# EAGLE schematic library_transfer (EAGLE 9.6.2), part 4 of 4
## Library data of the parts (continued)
U84 = ruark2:NCP781BMNADJTAGOSCT-ND: 150V 100mA Linear Voltage Regulator IC Positive Adjustable 1 Output 100mA 6-DFN (3.3x3.3); PARTNO: NCP781BMNADJTAGOSCT-ND
U85 = ruark2:NCP508SQ28T1G: Linear Voltage Regulator IC 1 Output 50mA SC-88A (SC-70-5/SOT-353); PARTNO: NCP508SQ28T1GOSCT-ND
U86 = ruark2:MTI-7-T: Accelerometer, Gyroscope, Magnetometer, 9 Axis Sensor I²C, SPI, UART Output; PARTNO: MTI-7-T-ND
U87 = ruark2:MPQ4436GRE-AEC1-Z: 45V 6A Buck Switching Regulator IC Positive Adjustable 0.815V 1 Output 20-PowerVFQFN; PARTNO: 1589-MPQ4436GRE-AEC1-ZCT-ND
U88 = ruark2:MP86952
U89 = ruark2:MP5515: Wide Input 2.7 - 18V, 5A, High-Efficiency Bidirectional, Power Back-Up Manager with Integrated Hot-Swap, I2C, ADC, and Cap Health Test
U90 = ruark2:MP3423: Boost Switching Regulator IC Positive Adjustable 2.5V 1 Output 9A (Switch) 14-PowerVFQFN; PARTNO: 1589-1171-1-ND
U91 = ruark2:MIC28516T-E/PHA: Switching Voltage Regulators 70V/8A Hyper Speed Control Synchronous DC/DC Buck Regulator with External Soft Start; PARTNO: 150-MIC28516T-E/PHACT-ND
U92 = ruark2:MIC7221YM5-TR: Comparator General Purpose Open Drain SOT-23-5; PARTNO: 576-2901-1-ND
U93 = ruark2:MIC4604YM-TR: Half-Bridge Gate Driver IC Non-Inverting 8-SOIC, 85V, 1A; PARTNO: 576-4396-1-ND
U94 = ruark2:MIC2920A-12WS: Linear Voltage Regulator IC Positive Fixed 1 Output 12V 400mA SOT-223; PARTNO: 576-1750-5-ND
U95 = ruark2:MIC2288: Boost Switching Regulator IC Positive Adjustable 2.5V 1 Output 1.2A (Switch) SOT-23-5 Thin, TSOT-23-5, IN 2.5-10, OUT 2.5-34; PARTNO: 576-1729-1-ND
U96 = ruark2:MIC2176-1YMM: Buck Regulator Positive Output Step-Down DC-DC Controller IC 10-MSOP 4.5-65V Synchronous; PARTNO: 576-3756-5-ND
U97 = ruark2:MIC842LYC5-TR: Comparator with Voltage Reference Push-Pull SC-70-5 Active High
U98 = ruark2:ME6211C12M5G-N: 300mA 70dB@(1kHz) Fixed 1.2V Positive electrode 6.5V SOT-23-5 Linear Voltage Regulators (LDO) ROHS; JLCPCB: C236672
U99 = ruark2:MCP73832T-5ACI/OT: Charger IC Lithium Ion/Polymer SOT-23-5 450mA; PARTNO: MCP73832T-5ACI/OTCT-ND
U100 = ruark2:MCP73811T-420I/OT: Charger IC Lithium Ion/Polymer SOT-23-5 450mA; PARTNO: MCP73811T-420I/OTCT-ND
U101 = ruark2:MCP73114-0NSI/MF: Charger IC Lithium Ion/Polymer 10-DFN (3x3); PARTNO: MCP73114-0NSI/MF-ND
U102 = ruark2:MCP23017: I/O Expander 16 CH, I²C 1.7MHz 28-SSOP; PARTNO: MCP23017T-E/SSCT-ND
U103 = ruark2:MCP9700: Temperature Sensor Analog, Local -40°C ~ 125°C 10mV/°C SOT-23-3; PARTNO: MCP9700T-E/TTCT-ND
U104 = ruark2:MCP6561T-E/OTVAO: Comparator General Purpose CMOS, Push-Pull, Rail-to-Rail, TTL SOT-23-5, 800ns, 5mVh; PARTNO: 150-MCP6561T-E/OTVAOCT-ND
U105 = ruark2:MCP6549-I/ST: Comparator General Purpose CMOS, 1uA power, 10pA bias, 7mV offset, Open-Drain, Rail-to-Rail, TTL 14-TSSOP; PARTNO: MCP6549-I/ST-ND
U106 = ruark2:MCP6542T-I/SN: Comparator General Purpose CMOS, Push-Pull, Rail-to-Rail, TTL 8-SOIC; PARTNO: MCP6542T-I/SNCT-ND
U107 = ruark2:MCP4725A1T-E/CH: 12 Bit Digital to Analog Converter 1 SOT-23-6 DAC I2C; PARTNO: MCP4725A1T-E/CHCT-ND
U108 = ruark2:MCP1702T-5002E/CB: Linear Voltage Regulator IC Positive Fixed 1 Output 250mA SOT-23A-3; PARTNO: MCP1702T-5002E/CBCT-ND
U109 = ruark2:MCP1665T-E/MRA: Boost Switching Regulator IC Positive Adjustable 2.8V 1 Output 1A 10-VFQFN Exposed Pad; PARTNO: MCP1665T-E/MRACT-ND
U110 = ruark2:MCP1632-BAE/MS: Boost, Cuk, Flyback, SEPIC Regulator Positive Output Step-Up, Step-Up/Step-Down DC-DC Controller IC 8-MSOP; PARTNO: MCP1632-BAE/MS-ND
U111 = ruark2:MCP1407-E/SN: Low-Side Gate Driver IC Non-Inverting 8-SOIC, 6A; PARTNO: MCP1407-E/SN-ND
U112 = ruark2:MCP6L01T-E/OT: General Purpose Amplifier 1 Circuit Rail-to-Rail SOT-23-5; PARTNO: MCP6L01T-E/OTCT-ND
U113 = ruark2:MC14044BDR2G: THIS PN HAS INVERED INPUTS S-R Latch 4 Channel 1:1 IC Tri-State 16-SOIC; PARTNO: MC14044BDR2GOSCT-ND
U114 = ruark2:MC14043BDR2G: IC LATCH R-S QUAD P/N 16-SOIC; PARTNO: MC14043BDR2GOSCT-ND
U115 = ruark2:MC74LVX08DTR2G: Quad 2-Input AND Gate AND Gate IC 4 Channel 14-TSSOP; MPN: MC74LVX08DTR2G; OC_FARNELL: 1353762; OC_NEWARK: 26K4279; PACKAGE: TSSOP-14; PARTNO: MC74LVX08DTR2GOSCT-ND; SUPPLIER: On Semiconductor
U116 = ruark2:MAX9107: Comparator General Purpose TTL 8-SOIC; PARTNO: MAX9107ESA+-ND
U117 = ruark2:MAX9095ASD+: Comparator General Purpose Open Drain 14-SOIC; PARTNO: MAX9095ASD+-ND
U118 = ruark2:MAX5084ATT+T: 65V Linear Voltage Regulator IC Positive Adjustable (Fixed) 1 Output 200mA 6-TDFN-EP (3x3); PARTNO: MAX5084ATT+CT-ND
U119 = ruark2:MAX3232ECDR: 3.3V 2/2 Transceiver Full RS232 16-SOIC; PARTNO: 296-19851-1-ND
U120 = ruark2:MAX2680AUT+T: RF Mixer IC Cellular, ISM, PCS, WLL Down Converter 400MHz ~ 2.5GHz SOT-23-6; PARTNO: MAX2680AUT+T-ND
U121 = ruark2:MAX2671EUT+T: RF Mixer IC Cellular, ISM, PCS, WLAN Up Converter 400MHz ~ 2.5GHz SOT-6; PARTNO: MAX2671EUT+TCT-ND
U122 = ruark2:MAX2663EUT+T: RF Mixer IC Cellular, ISM, PCS, WLAN Up Converter 400MHz ~ 2.5GHz SOT-23-6; PARTNO: MAX2663EUT+T-ND
U123 = ruark2:MAX232: 2/2 Transceiver Full RS232 16-SOIC; PARTNO: 296-26141-1-ND
U124 = ruark2:MAX-M8Q-0: MAX-M8 RF Receiver BeiDou, Galileo, GLONASS, GNSS, GPS 1.575GHz -167dBm; PARTNO: 672-MAX-M8Q-0CT-ND
U125 = ruark2:LTV827S-TA1: Optoisolator Transistor Output 5000Vrms 2 Channel 8-SMD; PARTNO: 160-2040-1-ND
U126 = ruark2:LTV-816S: Optoisolator Transistor Output 5000Vrms 1 Channel 4-SMD; PARTNO: 160-1892-1-ND
U127 = ruark2:LTC6993CS6-1#TRMPBF: Fixed Pulse Generator Monostable Multivibrator 11ns TSOT-23-6; PARTNO: LTC6993CS6-1#TRMPBFCT-ND
U128 = ruark2:LTC6992CS6-1#TRMPBF: Oscillator, Silicon IC 3.81Hz ~ 1MHz TSOT-23-6; PARTNO: LTC6992CS6-1#TRMPBFCT-ND
U129 = ruark2:LTC6990CS6#TRMPBF: VCO Oscillator, Silicon IC 488Hz ~ 1MHz TSOT-23-6; PARTNO: LTC6990CS6#TRMPBFCT-ND
U130 = ruark2:LTC4365: Overvoltage, Undervoltage and Reverse Supply Protection Controller Charge Pump, -40 to +60V
U131 = ruark2:LT8410IDC#TRMPBF: Boost Switching Regulator IC Positive Adjustable 1.235V 1 Output 20mA (Switch) 8-WFDFN Exposed Pad; PARTNO: LT8410IDC#TRMPBFCT-ND
U132 = ruark2:LT6654BHS6-2.5#TRMPBF: 2.5V Series Voltage Reference IC ±0.1% TSOT-23-6; PARTNO: LT6654BHS6-2.5#TRMPBFCT-ND
U133 = ruark2:LT3088EDD#PBF: Linear Voltage Regulator IC Positive Adjustable 36V 1 Output 800mA 8-DFN (3x3); PARTNO: LT3088EDD#PBF-ND
U134 = ruark2:LT3080: Linear Voltage Regulator IC Positive Adjustable 1 Output 0 V ~ 36 V 1.1A SOT-223-3; PARTNO: LT3080EST#TRPBFCT-ND
U135 = ruark2:LT3012EFETRPBF: 60V 250mA LDO Linear Voltage Regulator IC Positive Adjustable 1 Output 16-TSSOP-EP; PARTNO: LT3012EFE#TRPBFCT-ND
U136 = ruark2:LT1678: General Purpose Amplifier 2 Circuit Rail-to-Rail 8-SO 20MHz Rail to Rail; PARTNO: LT1678CS8#TRPBFCT-ND
U137 = ruark2:LT1054: Charge Pump Switching Regulator IC Positive or Negative Adjustable (Fixed) 3.5V (-Vin, 2Vin) 1 Output 100mA 16-SOIC (0.295", 7.50mm Width); PARTNO: 296-17595-1-ND
U138 = ruark2:LP28013A: TDFN-10 Battery Management ICs ROHS JLCPCB: C517139
U139 = ruark2:LMV7219M5X: Comparator General Purpose Push-Pull, Rail-to-Rail SOT-23-5 (OPA320 pinout compatible); PARTNO: LMV7219M5X-ND
U140 = ruark2:LMV321IDBVR: General Purpose Amplifier 1 Circuit Rail-to-Rail SOT-23-5; PARTNO: 296-9567-1-ND
U141 = ruark2:LMT87LPG: Temperature Sensor Analog, Local -50°C ~ 150°C 13.6mV/°C TO-92S; PARTNO: 296-47011-ND
U142 = ruark2:LMR38020SDDAR: Buck Switching Regulator IC Positive Adjustable 1V 1 Output 2A 8-PowerSOIC (0.154", 3.90mm Width); PARTNO: 296-LMR38020SDDARCT-ND
U143 = ruark2:LMP2231: General Purpose Amplifier 1 Circuit Rail-to-Rail SOT-23-5, 0.02pA, 10uV
U144 = ruark2:LMC7660: Charge Pump Switching Regulator IC Negative Fixed -Vin 1 Output 8-SOIC (0.154", 3.90mm Width); PARTNO: LMC7660IMX/NOPBCT-ND
U145 = ruark2:LMC662CN/NOPB: SURFACE MOUNT DIP SOCKET FOR: LMC662CN/NOPB CMOS Amplifier 2 Circuit Push-Pull, Rail-to-Rail 8-PDIP | PURCHASE 110-87-308-41-105191; PARTNO: LMC662CN/NOPB-ND
U146 = ruark2:LMC662CMX/NOPB: CMOS Amplifier 2 Circuit Push-Pull, Rail-to-Rail 8-SOIC; PARTNO: 296-36891-1-ND
U147 = ruark2:LMC555CMM/NOPB: 555 Type, Timer/Oscillator (Single) IC 2.1MHz 8-SOIC; PARTNO: LMC555CMM/NOPBCT-ND
U148 = ruark2:LM46002AQPWPRQ1: Buck Switching Regulator IC Positive Adjustable 1V 1 Output 2A 16-TSSOP (0.173", 4.40mm Width) Exposed Pad 60V; PARTNO: 296-48923-1-ND
U149 = ruark2:LM25116MHX/NOPB: Buck Regulator Positive Output Step-Down DC-DC Controller IC 20-HTSSOP; PARTNO: 296-35258-1-ND
U150 = ruark2:LM7301: General Purpose Amplifier 1 Circuit Rail-to-Rail SOT-23-5; PARTNO: LM7301IM5X/NOPBCT-ND
U151 = ruark2:LM5155: Boost, Flyback, SEPIC Regulator Positive Output Step-Up, Step-Up/Step-Down DC-DC Controller IC 12-WSON (3x2); PARTNO: 296-LM5155DSSRCT-ND
U152 = ruark2:LM5134-SOT: Low-Side Gate Driver IC Inverting, Non-Inverting SOT-23-6 7.6A; PARTNO: 296-40244-1-ND
U153 = ruark2:LM5102MM/NOPB: IC GATE DRVR HALF-BRIDGE 10VSSOP; PARTNO: LM5102MM/NOPBCT-ND
U154 = ruark2:LM4040DYM3-2.5-TR: Shunt Voltage Reference IC ±1% 15mA SOT-23-3; PARTNO: 576-1047-1-ND
U155 = ruark2:LAN9512: Ethernet Bridge, USB to Ethernet USB 2.0, 10/100 Base-T/TX PHY USB Interface 64-QFN (9x9); PARTNO: 638-1086-ND
U156 = ruark2:LAN8742A-CZ-TR: 1/1 Transceiver Ethernet 24-SQFN (4x4); PARTNO: LAN8742A-CZ-CT-ND
U157 = ruark2:L6491: Half-Bridge Gate Driver IC Non-Inverting 14-SO 4A; PARTNO: 497-15443-5-ND
U158 = ruark2:L5150BNTR: Linear Voltage Regulator IC 40 Vin Positive Output 5V 150mA SOT-223; PARTNO: 497-11659-1-ND
U159 = ruark2:L4931: Linear Voltage Regulator IC Positive Fixed 1 Output 5V 250mA 8-SO; PARTNO: 497-1156-1-ND
U160 = ruark2:L78M05ABDT-TR: 62dB@(120Hz) 500mA Fixed 5V Positive 35V TO-252 Linear Voltage Regulators (LDO) ROHS; PARTNO: C58069
U161 = ruark2:K78U05-500R3: Non-Isolated PoL Module DC DC Converter 1 Output 5V 500mA 9V - 90V Input; PARTNO: 2725-K78U05-500R3-ND
U162 = ruark2:ISO1640BDR: I²C Digital Isolator 3000Vrms 2 Channel 50kV/µs CMTI 8-SOIC (0.154", 3.90mm Width); PARTNO: 296-ISO1640BDRCT-ND
U163 = ruark2:ISL83490IBZ-T: 1/1 Transceiver Full RS422, RS485 8-SOIC 3.3V; PARTNO: ISL83490IBZ-TCT-ND
U164 = ruark2:ISL21080DIH312Z-TK: Series Voltage Reference IC 1.25V ±0.6% 7mA SOT-23-3; PARTNO: ISL21080DIH312Z-TKCT-ND
U165 = ruark2:IRS2304SPBF: Half-Bridge Gate Driver IC Non-Inverting 8-SOIC 600V 290mA; PARTNO: IRS2304SPBF-ND
U166 = ruark2:IRS2186: Half-Bridge Gate Driver IC Non-Inverting 8-SOIC; PARTNO: IRS2186SPBF-ND
U167 = ruark2:IRM-05-5: Enclosed AC DC Converters 1 Uitgang 5V 1A 85 ~ 305 VAC, 120 ~ 430 VDC Input; PARTNO: 1866-3027-ND
U168 = ruark2:INA240A3PW: –4-V to 80-V, Bidirectional, Ultra-Precise Current Sense Amplifier With Enhanced PWM Rejection
U169 = ruark2:INA210CIDCKR: Current Sense Amplifier 1 Circuit SC-70-6 200V/V; PARTNO: 296-48548-1-ND
U170 = ruark2:INA195AIDBVR: 100 V/V, 3%, 80V, Current Monitor Regulator High-Side SOT-23-5; PARTNO: 296-26067-1-ND
U171 = ruark2:INA181A3IDBVR: Current Sense Amplifier 1 Circuit Rail-to-Rail SOT-23-6; PARTNO: 296-47658-1-ND
U172 = ruark2:INA180A3IDBVR: Current Sense Amplifier 1 Circuit Rail-to-Rail SOT-23-5 High/Low side 100V/V; PARTNO: 296-47654-1-ND
U173 = ruark2:HTCC-AB01: HTCC-AB01
U174 = ruark2:HMC544A: RF Switch IC WiMax, WLAN SPDT 4GHz 50 Ohm SOT-26; PARTNO: 1127-3066-ND
U175 = ruark2:HMC385LP4E: VCO 2.25GHz ~ 2.5GHz 24-QFN (4x4); PARTNO: 1127-1357-ND
U176 = ruark2:HELTEC_WIFI_LORA_32_V3
U177 = ruark2:HEF4052B: Dual 4 Channel Analog Multiplexer; PARTNO: 1727-6411-1-ND
U178 = ruark2:HD3SS3412ARUAT: PCI Express® Switch IC 4 Channel 42-WQFN (3.5x9.0); PARTNO: 296-HD3SS3412ARUATCT-ND
U179 = ruark2:HCF4010YM013TR: Voltage Level Translator Unidirectional 6 Circuit 1 Channel 16-SO; PARTNO: 497-13665-1-ND
U180 = ruark2:GVA-84+: RF Amplifier IC CATV, DBS, LTE, MMDS, Wireless LAN 0Hz ~ 7GHz SOT-89; PARTNO: 3157-GVA-84+CT-ND
U181 = ruark2:FT232RL: USB Bridge, USB to UART USB 2.0 UART Interface 28-SSOP FTDI; PARTNO: 768-1007-1-ND
U182 = ruark2:FM2113: SOT-23-6 Battery Protection UVLO, OV, OC
U183 = ruark2:FAN3180: Low-Side Gate Driver IC Non-Inverting SOT-23-5 2A; PARTNO: FAN3180TSXCT-ND
U184 = ruark2:FAN3111ESX: 1.4A, Low-Side Gate Driver IC Non-Inverting SOT-23-5; PARTNO: FAN3111ESXCT-ND
U185 = ruark2:EL5171: Single Ended to Differential Amplifier 1 Circuit 8-SOIC; PARTNO: EL5171ISZ-ND
U186 = ruark2:DS1100Z-500: Delay Line IC Nonprogrammable 5 Tap 500ns 8-SOIC (0.154", 3.90mm Width); PARTNO: DS1100Z-500+-ND
U187 = ruark2:DS18S20: Temperature Sensor Digital, Local -55°C ~ 125°C 8 b TO-92-3; PARTNO: DS18S20+-ND
U188 = ruark2:DRV8231ADDAR: 33V, 3.7A, Bipolar Motor Driver NMOS PWM 8-SO PowerPad 2 H-BRIDGE; PARTNO: 296-DRV8231ADDARCT-ND
U189 = ruark2:DP83822IRHBR: 10/100 Ethernet PHY RGMII/RMII/MII; PARTNO: 296-44794-1-ND
U190 = ruark2:DP83TD510ERHBR: 1/1 Transceiver 10BASE-T1L IEEE 802.3 32-VQFN (5x5); PARTNO: 296-DP83TD510ERHBRCT-ND
U191 = ruark2:DAC5571IDBVR: 8 Bit Digital to Analog Converter 1 SOT-23-6; PARTNO: 296-38918-1-ND
U192 = ruark2:COM13025-48.000-T-TR: 48 MHz XO (Standard) HCMOS Oscillator 3.3V Enable/Disable 4-SMD, No Lead; PARTNO: 2151-COM13025-48.000-T-TRCT-ND
U193 = ruark2:CO32H4-25.000-33GDTST: 3.3V~3.3V ±50ppm 25MHz HCMOS SMD3225-4P Oscillators ROHS 4-SMD, No Lead
U194 = ruark2:CM108: CM108 USB Audio
U195 = ruark2:CD40257: Multiplexer 4 x 1:2 16-SOIC; PARTNO: 296-32875-5-ND
U196 = ruark2:CD74HC4017M96: Counter IC Counter, Decade 1 Element 10 Bit Positive Edge 16-SOIC 35MHz; PARTNO: 296-12808-1-ND
U197 = ruark2:CBTL02042ABQ,115: DisplayPort, PCIe, USB Switch IC 2 Channel 20-DHVQFN (4.5x2.5); PARTNO: 568-6676-1-ND
U198 = ruark2:BQ7790512PWR: 3-5S Stackable to 20S Battery protection IC. 2.8V to 4.175V; PARTNO: 296-50465-1-ND
U199 = ruark2:BQ24616
U200 = ruark2:BQ24171: Charger IC Lithium Ion/Polymer 24-VQFN (5.5x3.5); PARTNO: 296-41205-1-ND
U201 = ruark2:BNO080: Accelerometer, Gyroscope, Magnetometer, 9 Axis Sensor I²C, SPI, UART Output; PARTNO: 1888-1000-1-ND
U202 = ruark2:BMP280: Pressure Sensor 4.35PSI ~ 15.95PSI (30kPa ~ 110kPa) Absolute 16b 8-SMD; PARTNO: 828-1064-1-ND
U203 = ruark2:BGU8051: RF Amplifier IC GSM, LTE, W-CDMA 300MHz ~ 1.5GHz 8-HWSON (2x2); PARTNO: 568-BGU8051XCT-ND
U204 = ruark2:BGU6102,147: RF Amplifier 40MHz - 4GHz, P1dB =9.5dBm, G=19dB, NF=2.3dB, I=20mA, V=1.5-5V, 6-HXSON (1.3x2); PARTNO: 568-10150-1-ND
U205 = ruark2:BGB741L7ESDE6327XTSA1: RF Amplifier IC Cellular, RKE, WiFi 50MHz ~ 3.5GHz PG-TSLP-7-1, NF=1dB, P1dB= -6.6dBm; PARTNO: BGB741L7ESDE6327XTSA1CT-ND
U206 = ruark2:BGA2869,115: RF Amplifier IC General Purpose 0Hz ~ 2.2GHz 6-TSSOP; PARTNO: 568-8535-1-ND
U207 = ruark2:BGA2866,115: RF Amplifier 0Hz - 2.2GHz, P1dB=3dBm, G=24.3dB, NF=3.9, I=17.4mA, V=5V, 6-TSSOP; PARTNO: 568-6213-1-ND
U208 = ruark2:BGA427H6327XTSA1: RF Amplifier 0Hz - 3GHz, G=18.5 dB, NF= 2.2dB, I= 25mA, V=2-5V, PG-SOT343-4; PARTNO: BGA427H6327XTSA1CT-ND
U209 = ruark2:BD9C401EFJ-E2: Buck Switching Regulator IC Positive Adjustable 0.8V 1 Output 4A 8-SOIC (0.154", 3.90mm Width) Exposed Pad; PARTNO: 846-1116-1-ND
U210 = ruark2:B39921B2672P810: 915MHz Frequency General Purpose RF SAW Filter (Surface Acoustic Wave) 1.1dB 26MHz Bandwidth 5-SMD, No Lead; PARTNO: 1752-B39921B2672P810CT-ND
U211 = ruark2:B39431B3710U410: 433.92MHz Frequency Remote Control RF SAW Filter (Surface Acoustic Wave) 2dB 1.7MHz Bandwidth 6-SMD, No Lead
U212 = ruark2:AX5043: IC RF TxRx Only General ISM < 1GHz 27MHz ~ 1.05GHz 28-VFQFN Exposed Pad; PARTNO: AX5043-1-TA05OSCT-ND
U213 = ruark2:ATTINY85V-10SUR: AVR AVR® ATtiny, Functional Safety (FuSa) Microcontroller IC 8-Bit 10MHz 8KB (4K x 16) FLASH 8-SOIC; PARTNO: ATTINY85V-10SURCT-ND
U214 = ruark2:ATA6561-GAQW-N: 1/1 Transceiver CAN 8-SO; PARTNO: ATA6561-GAQW-NCT-ND
U215 = ruark2:AT2659: 1.4V~3.6V 4.3mA DFN-6(1x1.6) Low Noise Amplifiers (LNA) - RF ROHS; JLCPCB: C92450
U216 = ruark2:AP65550SP-13: Buck Switching Regulator IC Positive Adjustable 0.76V 1 Output 5A 8-SOIC (0.154", 3.90mm Width) Exposed Pad; PARTNO: AP65550SP-13DICT-ND
U217 = ruark2:AP9211SA: Battery Battery Protection IC Lithium-Ion U-DFN2030-6 (Type C); PARTNO: AP9211SA-AE-HAC-7DICT-ND
U218 = ruark2:AP2114H-3.3: Linear Voltage Regulator IC Positive Fixed 1 Output 3.3V 1A SOT-223; PARTNO: AP2114H-3.3TRG1DICT-ND
U219 = ruark2:AP2114H-2.5: Linear Voltage Regulator IC Positive Fixed 1 Output 2.5V 1A SOT-223; PARTNO: AP2114H-2.5TRG1DICT-ND
U220 = ruark2:AP2114H-1.8: Linear Voltage Regulator IC Positive Fixed 1 Output 1.8V 1A SOT-223; PARTNO: AP2114H-1.8TRG1DICT-ND
U221 = ruark2:AOZ128: Buck Switching Regulator IC Positive Adjustable 0.8V 1 Output 4A 8-SOIC (0.154", 3.90mm Width) Exposed Pad; PARTNO: 785-1689-1-ND
U222 = ruark2:AMS1117-3.3: 72dB@(120Hz) 1A Fixed 3.3V Positive electrode SOT-223-3 Linear Voltage Regulators (LDO) ROHS
U223 = ruark2:AG1170: Aliexpress SLIC
U224 = ruark2:ADS1115IDGSR: 16 Bit Analog to Digital Converter 2 Input 1 Sigma-Delta 10-VSSOP; PARTNO: 296-38849-1-ND
U225 = ruark2:ADP7142AUJZ-3.3-R7: 40V Linear Voltage Regulator IC Positive Fixed 3.3V 1 Output 200mA TSOT-23-5; PARTNO: ADP7142AUJZ-3.3-R7CT-ND
U226 = ruark2:ADG812YRUZ-REEL7: 4 Circuit IC Switch 1:1 650mOhm 16-TSSOP SPST; PARTNO: ADG812YRUZ-REEL7CT-ND
U227 = ruark2:ADF4351: IC SYNTH PLL VCO 32LFCSP; PARTNO: ADF4351BCPZ-RL7CT-ND
U228 = ruark2:ADF4118BRUZ: IC PLL FREQ SYNTHESIZER 16-TSSOP 3GHz; PARTNO: ADF4118BRUZ-ND
U229 = ruark2:AD8306: Limiting-Logarithmic Amplifier IC Receiver Signal Strength Indication (RSSI) 16-SO; PARTNO: AD8306ARZ-ND
U230 = ruark2:ACS781KLRTR-150B-T: Current Sensor 150A 1 Channel Hall Effect, Differential Bidirectional 7-PowerSMD Module. 3V3, 8.8mV/A; PARTNO: 620-1827-1-ND
U231 = ruark2:ACS711ELCTR-25AB-T: Current Sensor 25A 1 Channel Hall Effect, Open Loop Bidirectional 8-SOIC (0.154", 3.90mm Width); PARTNO: 620-1371-1-ND
U232 = ruark2:ACS711ELCTR-12AB-T: Current Sensor 12.5A 1 Channel Hall Effect, Open Loop Bidirectional 8-SOIC (0.154", 3.90mm Width), 5V; PARTNO: 620-1370-1-ND
U233 = ruark2:ACPL-782T-300E: Isolation Amplifier 1 Circuit Differential 8-DIP Gull Wing; PARTNO: 516-2337-5-ND
U234 = ruark2:0026605020: Connector Header Through Hole, Right Angle 2 position 0.156" (3.96mm); PARTNO: WM4640-ND
U235 = ruark2:74VHC4040FT: Counter IC Binary Counter 1 Element 12 Bit Negative Edge 16-TSSOP; PARTNO: 74VHC4040FTCT-ND
U236 = ruark2:74LVCH2T45DC,125: Voltage Level Translator Level Shifter Bidirectional 1 Circuit 2 Channel 420Mbps 8-VSSOP; PARTNO: 1727-4596-1-ND
U237 = ruark2:74LVC4245A: Voltage Level Translator Bidirectional 1 Circuit 8 Channel 24-TSSOP; PARTNO: 1727-4308-1-ND
U238 = ruark2:74HC4051D,653: 1 Circuit IC Switch 8:1 120Ohm 16-SO +/- 4V; PARTNO: 1727-2807-1-ND
U239 = ruark2:74AHC14PW,112: IC HEX SCHMITT-TRIG INV 14TSSOP; PARTNO: 296-1086-1-ND
U240 = ruark2:000: 1 Circuit IC Switch 8:1 75Ohm 16-SOIC; PARTNO: 296-3827-1-ND
U$1 = ruark2:ZF43610
U$2 = ruark2:XT30PW-F
U$3 = ruark2:WA-T247-101E: Heat Sink TO-247 Aluminum 1.0W @ 20°C Board Level, Vertical; PARTNO: WA-T247-101E-ND
U$4 = ruark2:VERT-55351
U$5 = ruark2:UA78M33CKVURG3: Linear Voltage Regulator IC 1 Output 500mA TO-252-3; PARTNO: 296-21208-1-ND
U$6 = ruark2:TRF37D73IDSGT: RF Amplifier IC 1MHz - 6GHz, P1dB=16.5dB, G=19.5dB, NF=3.2dB, 8-WSON (2x2); PARTNO: 296-38827-1-ND
U$7 = ruark2:TP65H035WS: N-Channel 650V 46.5A (Tc) 156W (Tc) Through Hole TO-247-3 WARNING: GATE-SOURCE-DRAIN!; PARTNO: TP65H035WS-ND
U$8 = ruark2:TOROID2
U$9 = ruark2:TOROID1
U$10 = ruark2:TDA21490
U$11 = ruark2:STW40N65M2: N-Channel 650V 32A (Tc) 250W (Tc) Through Hole TO-247; PARTNO: 497-15576-5-ND
U$12 = ruark2:SPU01M-05: Isolated Module DC DC Converter 1 Output 5V 200mA 10.8V - 13.2V Input; PARTNO: SPU01M-05
U$13 = ruark2:SP1312/S
U$14 = ruark2:SIP32408DNP-T1-GE4: Power Switch/Driver 1:1 N-Channel 3.5A 4-TDFN (1.2x1.6); PARTNO: SIP32408DNP-T1-GE4CT-ND
U$15 = ruark2:PLUG
U$16 = ruark2:PINHD20
U$17 = ruark2:PA1005.100NLT: 20A 1:100 Current Sense Transformer 50kHz ~ 1MHz 0.75 mOhm Primary, 5.5 Ohm Secondary 2mH Surface Mount; PARTNO: PA1005.100NLT
U$18 = ruark2:OLED
U$19 = ruark2:MC3417: Continuously Variable Slope Delta (CVSD) Modulator / Demodulator
U$20 = ruark2:LM25037: Full-Bridge, Half-Bridge, Push-Pull Regulator Positive, Isolation Capable Output Step-Up/Step-Down DC-DC Controller IC 16-TSSOP; PARTNO: 296-35257-1-ND
U$21 = ruark2:LM5134: Low-Side Gate Driver IC Inverting, Non-Inverting 6-WSON (3x3) 7.6A; PARTNO: 296-40245-1-ND
U$22 = ruark2:HMC313E: RF Amplifier IC HiperLAN, UNII, 0Hz - 6GHz, P1dB=14dBm, G=17dB, NF=6.5dB, I=50mA, V=5V, SOT-23-6; PARTNO: 1127-2932-ND
U$23 = ruark2:EPC2033: TRANS GAN 150V 7MOHM BUMPED DIE; PARTNO: 917-1131-1-ND
U$24 = ruark2:ECS-250-18-36B-CKY-TR: 25 MHz Crystal 10ppm; PARTNO: XC3051CT-ND
U$25 = ruark2:DS02C-254-1L-04BE: Dip Switch SPST 4 Position Through Hole, Right Angle Piano Actuator 25mA 24VDC; PARTNO: 2223-DS02C-254-1L-04BE-ND
U$26 = ruark2:CSAC
U$27 = ruark2:COUPLED_INDUCTOR2
U$28 = ruark2:COUPLED_INDUCTOR
U$29 = ruark2:CMZ5951CTR13: Zener Diode 120V 500mW ±5% Surface Mount SMA; PARTNO: CMZ5951BTR13CT-ND
U$30 = ruark2:BGA6589,135: RF Amplifier IC PCS, CDPD, Broadcast Television, 0Hz - 3GHz, P1dB=20dBm, G=17dB, NF=3.3dB, I=81mA, V=4.8V, SOT-89-3; PARTNO: 568-2075-1-ND
U$31 = ruark2:B38G3RGB-10D0003H2U1930: Red, Green, Blue (RGB) - LED Indication - Discrete 2V Red, 3V Green, 3V Blue 0606 (1616 Metric); PARTNO: 3147-B38G3RGB-10D0003H2U1930CT-ND
U$32 = ruark2:ADA4891-2ARZ-R7: General Purpose Amplifier 2 Circuit Rail-to-Rail 8-SOIC; PARTNO: ADA4891-2ARZ-R7CT-ND
U$33 = ruark2:AD8317: 8 GHz Logarithmic Amplifier IC Receiver Signal Strength Indication (RSSI) 8-LFCSP-VD (3x2); PARTNO: AD8317ACPZ-R7CT-ND
U$34 = ruark2:74439358010: 1µH Shielded Wirewound Inductor 17A 2.1 mOhm Nonstandard; PARTNO: 732-7273-1-ND
U$35 = ruark2:1841513: 4x2 Position Wire to Board Terminal Block Horizontal with Board 0.138" (3.50mm) Through Hole. Compatible with Cixi Kefa Elec KF207RH-3.5-2*4P; PARTNO: 277-10317-ND
U$36 = ruark2:100UH41A
U$37 = ruark2:100UH4A
U$38 = ruark2:10AWG: 10AWG Stranded Solder Hole
U$39 = ruark2:3:1TRANSFORMER
U$40 = ruark2:.42UH
V1 = ruark2:IV-6: Russian VFD Tube
VR1 = ruark2:ST4ETA104: 100 kOhms 0.25W, 1/4W J Lead Surface Mount Trimmer Potentiometer Cermet 1 Turn Top Adjustment; PARTNO: ST4ETA104CT-ND
VR2 = ruark2:ST4ETA102: 1 kOhms 0.25W, 1/4W J Lead Surface Mount Trimmer Potentiometer Cermet 1 Turn Top Adjustment; PARTNO: ST4ETA102CT-ND
VR3 = ruark2:PTV09A-4225F-B104: 100k Ohm 1 Gang Linear Through Hole, Snap In Potentiometer Detent 1 Turn Carbon 0.05W, 1/20W PC Pins, Board Locks (NOT RA); PARTNO: PTV09A-4225F-B104-ND
VR4 = ruark2:P160KN-0QC15B500K: 500k Ohm 1 Gang Linear Panel Mount Potentiometer None 1 Turn Conductive Plastic 0.2W, 1/5W PC Pins; PARTNO: 987-1304-ND
VR5 = ruark2:3224G-1-104E: 100 kOhms 0.25W, 1/4W Gull Wing Surface Mount Trimmer Potentiometer Cermet 12 Turn Side Adjustment; PARTNO: 3224G-1-104ECT-ND
X1 = ruark2:TA0862A: 1.26852GHz Frequency Wireless RF SAW Filter (Surface Acoustic Wave) 3.2dB 20.46MHz Bandwidth 6-SMD, No Lead; PARTNO: 4606-TA0862ACT-ND
X2 = ruark2:TA0289A: 159.0125MHz Frequency Wireless RF SAW Filter (Surface Acoustic Wave) 2.8dB 6.025MHz Bandwidth 10-SMD, No Lead; PARTNO: 5254-MA04627CT-ND
X3 = ruark2:SIT2024AA-S2-XXE-25.000000E: 25MHz XO (Standard) LVCMOS Oscillator 2.25V ~ 3.63V Enable/Disable SOT-23-5; PARTNO: 1473-SIT2024AA-S2-XXE-25.000000E-ND
X4 = ruark2:SIT2024AA-S2-XXE-8.000000E: 8MHz XO (Standard) LVCMOS Oscillator 2.25V ~ 3.63V Enable/Disable SOT-23-5; PARTNO: 1473-SIT2024AA-S2-XXE-8.000000E-ND
X5 = ruark2:RTX-2520AF333-S-32.000-TR: 32MHz TCXO Clipped Sine Wave Oscillator 3.3V 4-SMD, No Lead; PARTNO: 2151-RTX-2520AF333-S-32.000-TRCT-ND
X6 = ruark2:RTX-2520AF3F-S-10.000-TR: 10MHz TCXO Clipped Sine Wave Oscillator 4-SMD, No Lead, 500ppb; PARTNO: RTX-2520AF3F-S-10.000-TR
X7 = ruark2:NX2016SA-32M-EXS00A-CS06465: 32MHz Crystal 10pF 60 Ohms 4-SMD, No Lead; PARTNO: 644-1300-1-ND
X8 = ruark2:FC-13532.7680KA-AC0: 32.768kHz ±20ppm Crystal 9pF 70 kOhms 2-SMD, No Lead; PARTNO: SER4084CT-ND
X9 = ruark2:F6HH2G350EH75-J: 2.35GHz Frequency LTE, SCDMA RF SAW Filter (Surface Acoustic Wave) 1.4dB Bandwidth 5-SMD, No Lead; PARTNO: 587-F6HH2G350EH75-JCT-ND
X10 = ruark2:DSC1124DI5-390.0250T: 390.025 MHz XO (Standard) HCSL Oscillator 2.25V ~ 3.6V Enable/Disable 6-VDFN; PARTNO: 150-DSC1124DI5-390.0250T-ND
X11 = ruark2:ABM8-30.000MHZ-10-1-U-T: 30MHz ±10ppm Crystal 10pF 40 Ohms 4-SMD, No Lead; PARTNO: 535-9680-1-ND
X12 = ruark2:ABLS-12.000MHZ-B2-T: 12MHz ±20ppm Crystal 18pF 50 Ohms HC-49/US; PARTNO: 535-9067-1-ND
X13 = ruark2:ABLS-8.000MHZ-B4-T: 8MHz ±30ppm Crystal 18pF 80 Ohms HC-49/US; PARTNO: 535-10212-1-ND
X14 = ruark2:ABLS-6.000MHZ-20-B-3-H-T: 6MHz ±25ppm Crystal 20pF 100 Ohms HC-49/US; PARTNO: 535-14932-1-ND
X15 = ruark2:ABLS-4.000MHZ-B2-T: 4 MHz ±20ppm Crystal 18pF 180 Ohms HC-49/US; PARTNO: 535-9085-1-ND
Z1 = ruark2:ADE-25MH+: SMT Triple Balanced Mixer, RF/LO Freq 5 - 2500 MHz; PARTNO: 3157-ADE-25MH+CT-ND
